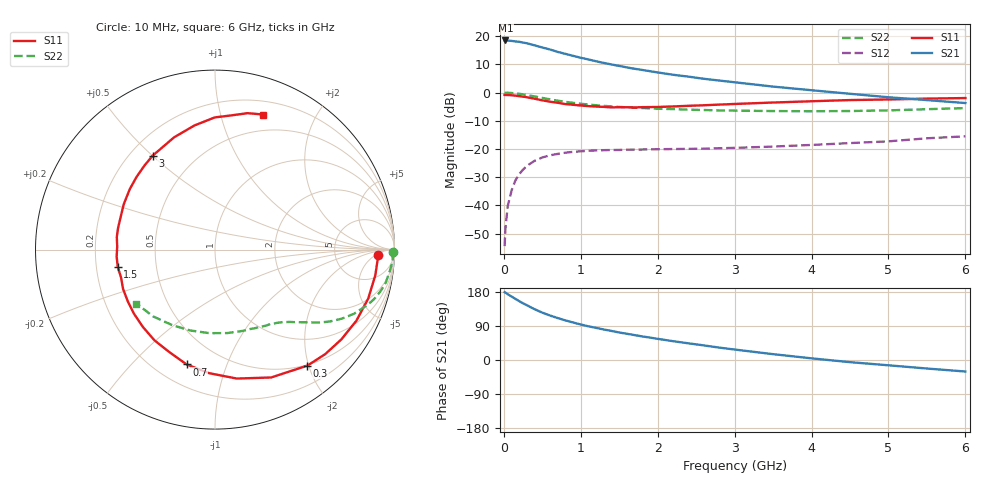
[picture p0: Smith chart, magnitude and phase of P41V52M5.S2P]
! SIEMENS Small Signal Semiconductors
! BFP182
! Si NPN RF Bipolar Junction Transistor in SOT143
! VCE = 1.5 V  IC = 2.5 mA
! Common Emitter S-Parameters:  March  1996
# GHz  S  MA  R  50
!  f  S11  S21  S12  S22
! GHz  MAG  ANG  MAG  ANG  MAG  ANG  MAG  ANG
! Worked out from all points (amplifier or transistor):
!   36 points, 10 MHz to 6 GHz, reference 50 ohm
!   highest |S21| = 18.5 dB at 20 MHz (marker M1)
!   |S21| within 3 dB of that: start of sweep to 571.6 MHz
!   unconditionally stable (mu >= 1): 1.994 GHz to end of sweep
!   at 250 MHz: K = 0.15, MSG = 22.5 dB, |S12| = -27.3 dB
!   at 1.4 GHz: K = 0.75, MSG = 15.2 dB, |S12| = -20.4 dB
!   at 6 GHz: K = 1.01, MAG = 5.3 dB, |S12| = -15.5 dB
!   S11 on the Smith chart (normalised r, x): 10 MHz: 19, -6; 300 MHz: 0.49, -1.98; 700 MHz: 0.32, -0.73; 1.5 GHz: 0.29, -0.08; 3 GHz: 0.29, +0.50; 6 GHz: 0.33, +1.37
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0.01  0.9085 -1.8  8.331 179.0  0.0019 84.9  0.9943 -0.7
0.02  0.9078 -3.6  8.376 178.0  0.0038 92.2  0.9892 -1.4
0.05  0.9045 -9.1  8.329 173.7  0.0097 86.0  0.9924 -3.6
0.1  0.8963 -17.7  8.226 167.5  0.0183 80.2  0.9805 -7.2
0.2  0.8637 -35.4  7.923 155.3  0.0359 70.4  0.9517 -14.0
0.25  0.8463 -43.5  7.697 149.5  0.0432 65.2  0.9283 -17.3
0.3  0.8262 -51.5  7.464 144.4  0.0504 61.3  0.9032 -20.0
0.4  0.7781 -66.3  6.861 134.0  0.0618 54.0  0.8541 -24.7
0.5  0.7286 -80.4  6.283 125.0  0.0708 47.6  0.8041 -28.6
0.6  0.6891 -92.8  5.795 117.4  0.0773 42.3  0.757 -31.9
0.7  0.659 -103.9  5.249 110.7  0.0819 38.1  0.7177 -34.4
0.9  0.6078 -123.7  4.471 99.0  0.0891 31.2  0.6569 -38.0
1.1  0.5756 -141.7  3.862 88.8  0.0931 26.4  0.6133 -41.2
1.3  0.5572 -156.8  3.349 80.5  0.0953 22.9  0.5808 -43.9
1.5  0.5504 -170.0  2.964 72.6  0.0962 20.7  0.5563 -46.5
1.8  0.5515 172.7  2.515 62.2  0.098 18.6  0.5319 -50.3
2.2  0.5677 153.6  2.066 49.6  0.0999 16.7  0.5095 -56.4
3  0.6281 123.6  1.522 27.6  0.1048 16.6  0.4789 -71.0
3.5  0.6659 110.0  1.275 15.4  0.1105 17.1  0.4701 -81.7
4.5  0.7365 90.1  0.951 -5.7  0.1273 17.4  0.4709 -106.7
5.5  0.7814 76.6  0.735 -22.5  0.1548 15.7  0.5074 -132.8
6  0.7994 70.3  0.652 -30.4  0.1678 12.4  0.5309 -145.5
